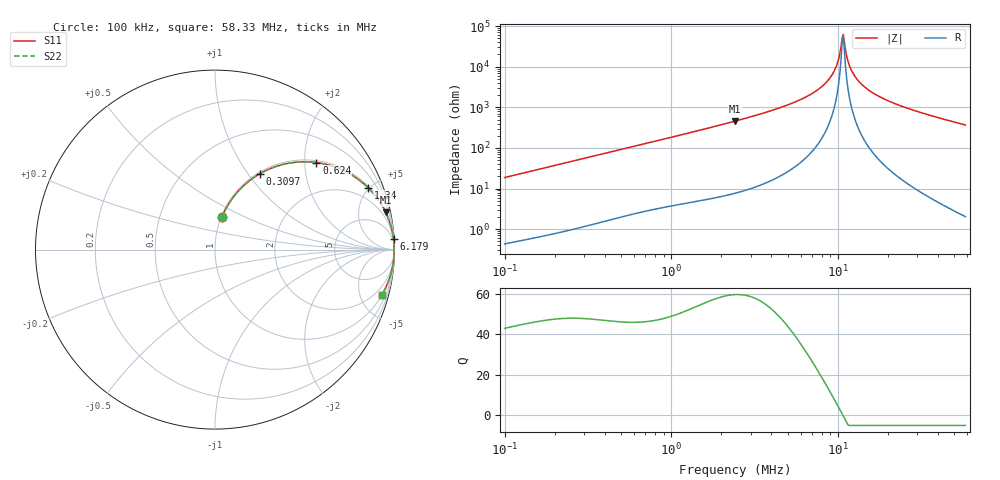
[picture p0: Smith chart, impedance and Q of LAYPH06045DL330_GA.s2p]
! LAYPH06045DL330_GA  S-PARAMETER MODEL  ( General Type )
! Model Generated by TAIYO YUDEN Corporation (http://www.ty-top.com)
! Version 2.0
! TAIYO YUDEN Control No. 180914NI43SB-FBB
! Copyright(c) 2018 TAIYO YUDEN CO.,LTD. All Rights Reserved.
! Product Description (link to TY-COMPAS)
! https://ds.yuden.co.jp/TYCOMPAS/or/detail?pn=LAYPH06045DL330MGA&u=M
! Products Name : Inductors
! Characteristics :
!  Inductance : 33 uH , SRF(min) : -Hz , DC Resistance(max) : 0.12 Ohm
!  Rated Current : Saturation :1.1 A , Temp Rise : 0.95 A (25 degC)
!  Case Size : 6.3 x 6.0 / 0.248 x 0.236 [mm/inch] , Thickness : 4.5 / 0.177 [mm/inch]
!  (Conditions: Temperature = 25 degC , DC Bias Current/Voltage = 0A / 0V)
! External Node Assignments :
!  1  o---GGG---o  2
! GND o---------o GND
! Frequency Range : 0.1MHz  -  58.334721MHz  [ 402 STEP ]
# MHz S RI R 50
! Freq[MHz].  S11 Real  S11 Imag  S21 Real  S21 Imag  S12 Real  S12 Imag  S22 Real  S22 Imag
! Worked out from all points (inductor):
!   401 points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, 100 kHz to 58.33 MHz, reference 50 ohm
!   read as one part in series: L = 29.6 uH near 103.2 kHz
!   highest Q = 59.7 at 2.415 MHz (marker M1), where L = 30.1 uH
!   self-resonance near 10.62 MHz
!   S11 on the Smith chart (normalised r, x): 100 kHz: 1.01, +0.37; 309.7 kHz: 1.02, +1.14; 624 kHz: 1.05, +2.29; 1.34 MHz: 1.09, +4.92; 6.179 MHz: 2, +33; 58.33 MHz: 1.04, -7.35
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0.1  0.0376 0.1791  0.9624 -0.1791  0.9624 -0.1791  0.0376 0.1791
0.290598  0.2286 0.4096  0.7714 -0.4096  0.7714 -0.4096  0.2286 0.4096
0.309708  0.251 0.4233  0.749 -0.4233  0.749 -0.4233  0.251 0.4233
0.624028  0.5654 0.485  0.4346 -0.485  0.4346 -0.485  0.5654 0.485
0.844473  0.7008 0.4474  0.2992 -0.4474  0.2992 -0.4474  0.7008 0.4474
1.340032  0.8535 0.3443  0.1465 -0.3443  0.1465 -0.3443  0.8535 0.3443
2.415258  0.9513 0.2071  0.0487 -0.2071  0.0487 -0.2071  0.9513 0.2071
2.454022  0.9528 0.2039  0.0472 -0.2039  0.0472 -0.2039  0.9528 0.2039
6.179279  0.9946 0.0599  0.0054 -0.0599  0.0054 -0.0599  0.9946 0.0599
7.018695  0.9962 0.0453  0.00376 -0.0453  0.00376 -0.0453  0.9962 0.0453
8.230089  0.9976 0.0279  0.00241 -0.0279  0.00241 -0.0279  0.9976 0.0279
9.200433  0.9981 0.0161  0.00185 -0.0161  0.00185 -0.0161  0.9981 0.0161
9.80545  0.9983 0.00947  0.00166 -0.00947  0.00166 -0.00947  0.9983 0.00947
10.45025  0.9984 0.00287  0.00156 -0.00287  0.00156 -0.00287  0.9984 0.00287
10.78838  0.9985 -0.000426  0.00155 0.000426  0.00155 0.000426  0.9985 -0.000426
10.96153  0.9985 -0.00207  0.00155 0.00207  0.00155 0.00207  0.9985 -0.00207
11.49783  0.9984 -0.00702  0.00158 0.00702  0.00158 0.00702  0.9984 -0.00702
11.86985  0.9984 -0.0103  0.00163 0.0103  0.00163 0.0103  0.9984 -0.0103
13.05973  0.9981 -0.0203  0.00192 0.0203  0.00192 0.0203  0.9981 -0.0203
15.55956  0.997 -0.0391  0.00302 0.0391  0.00302 0.0391  0.997 -0.0391
20.39619  0.9935 -0.0706  0.00648 0.0706  0.00648 0.0706  0.9935 -0.0706
58.33472  0.9299 -0.2526  0.0701 0.2526  0.0701 0.2526  0.9299 -0.2526
